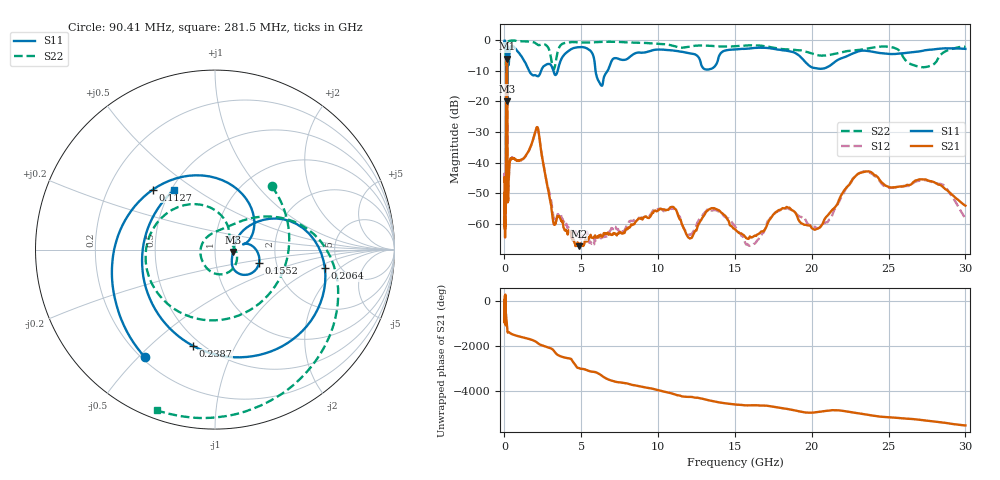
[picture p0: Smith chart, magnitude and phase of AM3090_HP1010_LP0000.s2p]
! Date/Time: Thu, Feb 28, 2019 2:04 PM
! Network Analyzer: Agilent Technologies E8364B Rev: A.07.50.67
! Sweep from 0.010 to 30.000 GHz, 1601 Points, Sweep Type: LOG
! Power Supply: 5.023 V, 0.002 A
# Hz S DB R 50
!freq MagS11 AngS11 MagS21 AngS21 MagS12 AngS12 MagS22 AngS22
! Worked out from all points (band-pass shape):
!   1601 points, 10 MHz to 30 GHz, reference 50 ohm
!   highest |S21| = -6.08 dB at 147.6 MHz (marker M1); lowest = -67.2 dB at 4.83 GHz (marker M2)
!   |S21| within 3 dB of the highest: 125.6 MHz to 177.6 MHz (51.98 MHz wide, 34.3 % of centre)
!   lowest |S11| = -19.9 dB at 181.3 MHz (marker M3), VSWR 1.22, Z = 61.1 - j1.57 ohm
!   |S11| at or under -10 dB: 1.604 GHz to 2.384 GHz (780.4 MHz wide, 39.1 % of centre); 3.184 GHz to 3.465 GHz (281 MHz wide, 8.45 % of centre); 5.927 GHz to 6.713 GHz (786.1 MHz wide, 12.4 % of centre)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
!   |S22| runs from -22.1 to -0.1 dB; largest |S21 - S12| = 0.012
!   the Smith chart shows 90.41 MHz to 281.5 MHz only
!   S11 on the Smith chart (normalised r, x): 90.41 MHz: 0.21, -0.52; 112.7 MHz: 0.40, +0.35; 155.2 MHz: 1.62, -0.27; 206.4 MHz: 3.81, -1.28; 238.7 MHz: 0.45, -0.69; 281.5 MHz: 0.52, +0.41
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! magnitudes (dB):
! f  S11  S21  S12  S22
! 10 MHz  -0.2  -46.2  -44.9  -0.5
! 38.04 MHz  -0.5  -59.7  -61.0  -1.2
! 47.41 MHz  -0.7  -49.4  -47.9  -1.5
! 90.41 MHz  -2.9  -54.1  -53.4  -6.5
! 112.7 MHz  -6.3  -21.5  -21.6  -8.0
! 144.7 MHz  -13.6  -6.1  -6.1  -18.3
! 147.6 MHz  -12.8  -6.1  -6.0  -17.5
! 155.2 MHz  -11.8  -6.2  -6.2  -16.7
! 181.3 MHz  -19.9  -10.7  -10.6  -16.8
! 206.4 MHz  -4.1  -48.3  -47.1  -2.5
! 238.7 MHz  -5.2  -52.5  -51.0  -0.8
! 281.5 MHz  -7.9  -44.4  -45.1  -0.4
! 550.5 MHz  -2.1  -38.5  -38.5  -0.2
! 2.084 GHz  -11.7  -28.7  -28.7  -1.2
! 3.204 GHz  -10.3  -59.9  -57.9  -9.6
! 4.83 GHz  -2.4  -67.2  -63.9  -0.8
! 6.234 GHz  -14.3  -63.6  -64.3  -0.6
! 7.926 GHz  -6.3  -61.7  -60.8  -0.8
! 13.61 GHz  -9.0  -54.8  -55.4  -1.9
! 16.21 GHz  -2.6  -64.0  -66.5  -1.7
! 23.48 GHz  -3.5  -42.9  -42.9  -2.9
! 30 GHz  -2.9  -54.0  -58.2  -2.2
